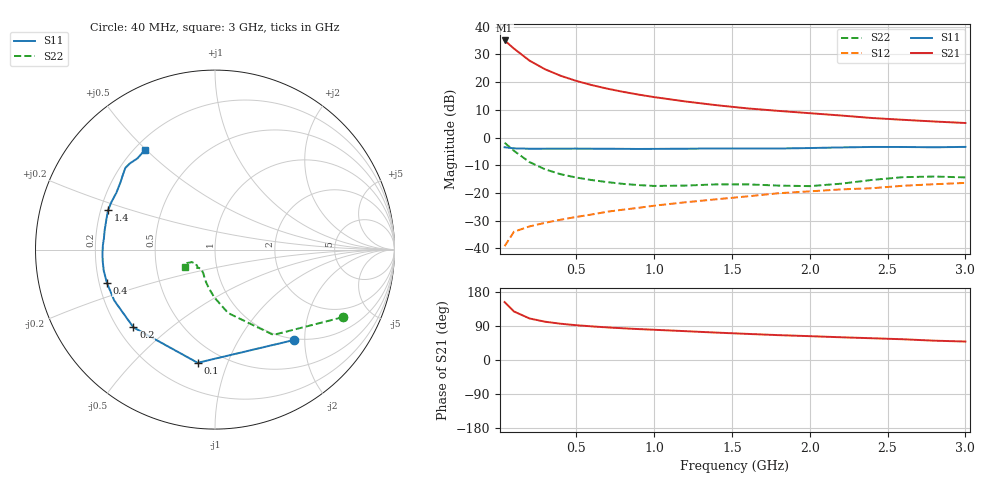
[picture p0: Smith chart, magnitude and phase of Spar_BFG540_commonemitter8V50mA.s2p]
! Filename:  BFG540L.S2P  Version:  3.0
! NXP part #: BFG540  Date: Feb 1992
! Bias condition: Vce=8V, Ic=50mA
! IN LINE PINNING: same data as with cross emitter pinning.
#  MHz  S  MA  R  50
! Freq  S11  S21  S12  S22  !GUM [dB]
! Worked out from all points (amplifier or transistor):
!   21 points, 40 MHz to 3 GHz, reference 50 ohm
!   highest |S21| = 35.0 dB at 40 MHz (marker M1)
!   |S21| within 3 dB of that: start of sweep to 101.7 MHz
!   unconditionally stable (mu >= 1): 705.4 MHz to end of sweep
!   at 300 MHz: K = 0.67, MSG = 27.7 dB, |S12| = -30.8 dB
!   at 1 GHz: K = 1.12, MAG = 17.5 dB, |S12| = -24.6 dB
!   at 3 GHz: K = 1.17, MAG = 8.3 dB, |S12| = -16.4 dB
!   S11 on the Smith chart (normalised r, x): 40 MHz: 0.97, -1.77; 100 MHz: 0.37, -0.79; 200 MHz: 0.26, -0.38; 400 MHz: 0.23, -0.14; 1.4 GHz: 0.23, +0.17; 3 GHz: 0.24, +0.49
40  0.668 -49.0  56.2 152.8  0.011 68.1  0.805 -27.9
100  0.638 -98.7  40.13 128.1  0.02 51.1  0.576 -55.6
200  0.628 -136.4  24.34 109.6  0.025 45.6  0.361 -78.3
300  0.629 -153.2  16.98 101.0  0.029 46.7  0.267 -90.7
400  0.63 -162.7  12.98 95.7  0.033 49.8  0.218 -99.0
500  0.631 -169.2  10.49 91.8  0.037 52.5  0.19 -104.9
600  0.629 -174.2  8.814 88.7  0.041 55.7  0.171 -109.5
700  0.627 -178.5  7.593 86.0  0.046 57.7  0.157 -113.2
800  0.625 177.7  6.67 83.7  0.05 59.5  0.146 -116.8
900  0.622 174.1  5.941 81.6  0.054 61.2  0.139 -120.9
1000  0.624 170.6  5.357 79.8  0.059 62.5  0.134 -124.9
1200  0.628 164.6  4.474 76.1  0.068 64.1  0.136 -131.6
1400  0.635 159.8  3.829 72.3  0.077 64.6  0.143 -134.1
1600  0.635 155.3  3.35 68.9  0.087 66.1  0.143 -134.2
1800  0.634 150.1  3.02 65.6  0.099 65.7  0.136 -136.3
2000  0.646 144.7  2.745 62.9  0.107 66.1  0.133 -143.6
2200  0.663 140.5  2.495 60.0  0.116 65.6  0.147 -151.8
2400  0.676 137.6  2.247 57.4  0.122 66.2  0.172 -154.3
2600  0.675 134.7  2.086 54.7  0.135 65.1  0.193 -151.8
2800  0.667 130.4  1.944 51.0  0.144 62.9  0.198 -148.9
3000  0.678 125.4  1.827 48.7  0.152 63.3  0.191 -150.3
